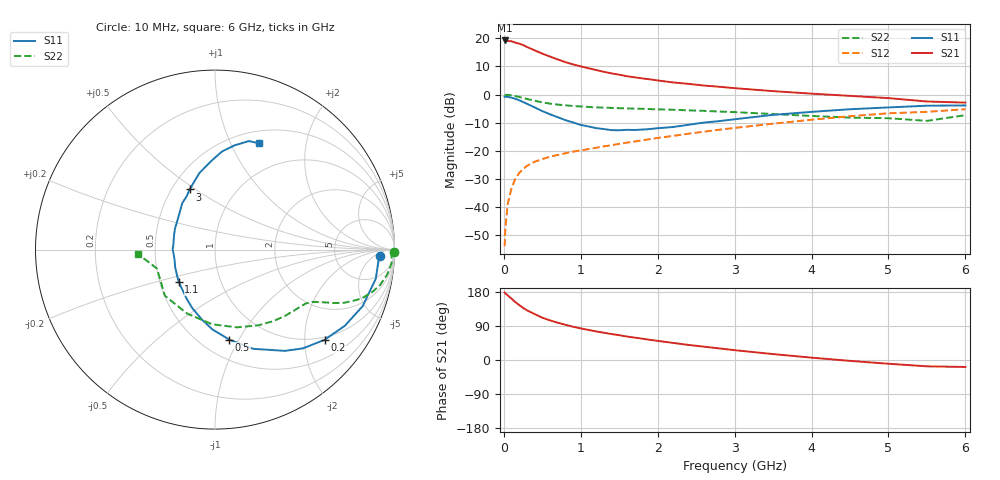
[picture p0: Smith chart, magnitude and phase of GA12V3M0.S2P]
! Infineon Technologies  Discrete & RF Semiconductors
! BF775
! Si NPN RF Bipolar Junction Transistor in SOT23
! VCE = 12 V  IC = 3 mA
! Common Emitter S-Parameters:  May  1996
# GHz  S  MA  R  50
!  f  S11  S21  S12  S22
! GHz  MAG  ANG  MAG  ANG  MAG  ANG  MAG  ANG
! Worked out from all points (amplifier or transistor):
!   36 points, 10 MHz to 6 GHz, reference 50 ohm
!   highest |S21| = 19.3 dB at 10 MHz (marker M1)
!   |S21| within 3 dB of that: start of sweep to 357.4 MHz
!   unconditionally stable (mu >= 1): 1.07 GHz to 3.031 GHz
!   at 250 MHz: K = 0.35, MSG = 22.1 dB, |S12| = -26.5 dB
!   at 1.4 GHz: K = 1.10, MAG = 10.9 dB, |S12| = -18.0 dB
!   at 6 GHz: K = 0.89, MSG = 1.2 dB, |S12| = -5.2 dB
!   S11 on the Smith chart (normalised r, x): 10 MHz: 20, -9; 200 MHz: 0.93, -2.48; 500 MHz: 0.68, -0.91; 1.1 GHz: 0.63, -0.24; 3 GHz: 0.61, +0.47; 6 GHz: 0.64, +1.29
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0.01  0.9184 -2.1  9.192 178.0  0.002 87.1  0.9962 -0.8
0.02  0.9127 -4.1  9.047 175.8  0.0042 84.4  0.9837 -1.7
0.05  0.9103 -10.3  9.002 170.7  0.0112 84.4  0.9873 -4.3
0.1  0.8808 -21.0  8.895 161.8  0.0216 78.5  0.9685 -8.4
0.15  0.8386 -30.4  8.405 152.7  0.0319 72.9  0.9407 -12.1
0.2  0.7908 -39.5  8.066 145.0  0.0402 68.5  0.9076 -15.1
0.25  0.7363 -48.4  7.613 137.5  0.0473 64.7  0.8695 -17.8
0.3  0.6854 -55.4  7.049 131.3  0.0537 62.1  0.835 -19.7
0.4  0.5921 -69.0  6.133 121.2  0.0636 57.6  0.7778 -22.4
0.5  0.5075 -81.0  5.353 111.6  0.0711 55.3  0.7269 -24.2
0.6  0.4454 -91.8  4.75 104.5  0.0784 53.8  0.6897 -25.3
0.8  0.3507 -110.9  3.781 92.9  0.0903 52.8  0.6431 -27.0
0.9  0.3188 -119.2  3.441 87.8  0.0963 53.1  0.6264 -27.7
1.1  0.2703 -138.5  2.945 79.4  0.1072 54.0  0.6017 -29.4
1.3  0.2432 -155.9  2.544 71.9  0.1198 54.7  0.5848 -31.3
1.6  0.2359 179.5  2.121 61.9  0.1394 55.5  0.5672 -34.8
2.2  0.2645 142.5  1.645 45.1  0.1839 55.6  0.5369 -43.7
3  0.3635 112.9  1.301 25.9  0.2548 51.9  0.4867 -60.1
3.5  0.4355 101.5  1.151 15.6  0.3031 47.8  0.4501 -74.2
4.5  0.5483 85.9  0.948 -2.3  0.4123 36.7  0.3887 -113.8
5.5  0.6333 72.7  0.753 -16.7  0.4926 20.6  0.3401 -161.9
6  0.6411 67.4  0.719 -18.4  0.5487 16.2  0.4294 -176.7
